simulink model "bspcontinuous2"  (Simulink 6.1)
settings: Solver=ode45  StartTime=0.0  StopTime=25  FixedStep=0.01  RelTol=1e-3
libraries: simulink x1

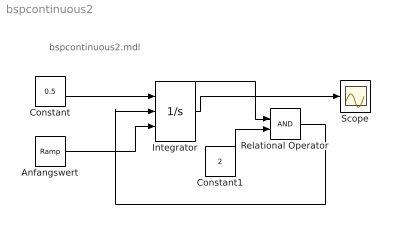
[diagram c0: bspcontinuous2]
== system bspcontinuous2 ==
  note: bspcontinuous2.mdl
  Anfangswert : simulink/Sources/Ramp  slope=0.1  start=0  X0=0
  Constant : Constant  Value=0.5
  Constant1 : Constant  Value=2
  Integrator : Integrator  ExternalReset=rising  InitialConditionSource=external  LimitOutput=on  UpperSaturationLimit=2  ShowStatePort=on
  Relational Operator : RelationalOperator
  Scope : Scope
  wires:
  Constant/1 -> Integrator/1
  Constant1/1 -> Relational Operator/2
  Anfangswert/1 -> Integrator/3
  Relational Operator/1 -> Integrator/2
  Integrator/1 -> Scope/1
  Integrator/State -> Relational Operator/1
